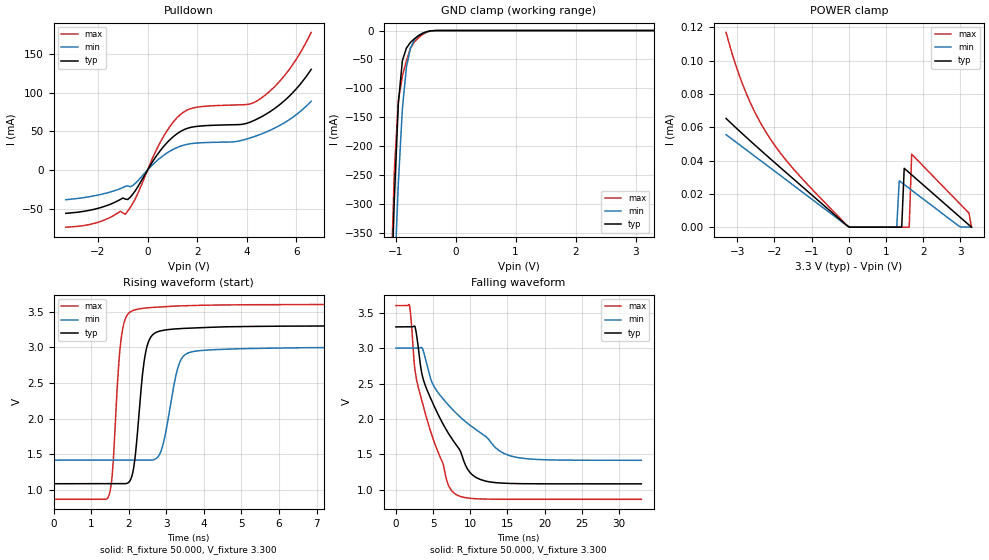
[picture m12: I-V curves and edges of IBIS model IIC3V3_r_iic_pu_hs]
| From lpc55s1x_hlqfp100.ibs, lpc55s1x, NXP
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|   Model IIC3V3_r_iic_pu_hs
[Model] IIC3V3_r_iic_pu_hs
Model_type I/O_open_drain
Polarity   Non-Inverting
Enable   Active-Low
Vinl =  0.990V
Vinh =  2.310V
Vmeas =  1.650V
Cref =  0.0F
Rref =  100.000
Vref =  3.3V
C_comp   2.434pF   2.433pF   2.440pF
C_comp_pulldown   1.615pF   1.554pF   1.667pF
C_comp_power_clamp   0.538pF   0.435pF   0.627pF
[Model Spec]
Vinh   2.310V   2.100V   2.520V
Vinl   0.990V   0.900V   1.080V
Vmeas   1.650V   1.500V   1.800V
Vref   3.3V   3.0V   3.6V
Cref   0.0F   0.0F   0.0F
Rref   100.000   100.000   100.000
[Temperature Range]   25.000   0.125k   -40.000
[Voltage Range]   3.300V   3.000V   3.600V
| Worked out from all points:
|   slope of the pulldown table from 0 to 0.495 V, typ, clamps not added: 20.4 ohm
|   GND clamp passes 1 mA (typ) near -0.43 V on its own axis
|   rising waveform, R_fixture 50.000, V_fixture 3.300: 20-80 % time 242ps typ, 336ps min, 194ps max; typ from 1.08 V to 3.3 V
|   falling waveform, R_fixture 50.000, V_fixture 3.300: 20-80 % time 5.56ns typ, 7.92ns min, 3.88ns max; typ from 3.3 V to 1.08 V
[Pulldown]
|Voltage   I(typ)   I(min)   I(max)
-3.3V     -56mA      -38.4mA    -73.87mA
-2.1V     -50.37mA   -33.07mA   -68.52mA
-1.1V     -38.15mA   -24.11mA   -53.37mA
-900mV    -37.61mA   -21.16mA   -57.18mA
-500mV    -26.92mA   -17.4mA    -37.43mA
500mV     24.51mA    15.34mA    35.14mA
1.2V      47.07mA    29.16mA    67.89mA
1.9V      55.94mA    34.55mA    80.54mA
3.8V      58.93mA    38.31mA    84.23mA
4.5V      67.15mA    45.39mA    91.04mA
5.6V      91.85mA    62.59mA    125mA
6.6V      130mA      88.72mA    177.8mA
[GND_clamp]
|Voltage   I(typ)   I(min)   I(max)
-3.3V     -10.05A    -9.18A     -11.33A
-1.089V   -516.5mA   -633.7mA   -475mA
-1.022V   -291.9mA   -436.3mA   -243.2mA
-955mV    -126mA     -264mA     -120.7mA
-888mV    -52.17mA   -135.6mA   -79.12mA
-821mV    -30.44mA   -63.69mA   -52.12mA
-754mV    -20.67mA   -30.69mA   -31.05mA
-687mV    -14.19mA   -15.97mA   -19.65mA
-553mV    -5.021mA   -4.512mA   -7.044mA
-419mV    -659.6uA   -714.3uA   -896.4uA
-285mV    -20.38uA   -37.42uA   -22.84uA
3.3V      0A         0A         0A
[POWER_clamp]
|Voltage   I(typ)   I(min)   I(max)
-3.3V     65.36uA    55.62uA    117.1uA
-2.797V   54.84uA    47.15uA    82.63uA
-2.194V   42.78uA    37.02uA    55.95uA
-50mV     976.9nA    858.9nA    1.15uA
1.29V     0A         0A         0A
1.357V    0A         27.85uA    0A
1.424V    0A         26.71uA    0A
1.491V    35.37uA    25.58uA    0A
1.625V    32.75uA    23.31uA    0A
1.692V    31.44uA    22.17uA    43.84uA
3.233V    1.309uA    0A         8.433uA
3.3V      0A         0A         0A
[Ramp]
| variable   typ   min   max
dV/dt_r   1.329/0.241n   0.951/0.336n   1.640/0.194n
dV/dt_f   1.329/5.558n   0.950/7.919n   1.640/3.880n
R_load = 50.000
[Rising Waveform]
R_fixture= 50.000
V_fixture= 3.300
V_fixture_min= 3.000
V_fixture_max= 3.600
|time   V(typ)   V(min)   V(max)
0s        1.085V     1.415V     866.6mV
1.467ns   1.085V     1.415V     908.4mV
1.83ns    1.084V     1.415V     3.23V
2.113ns   1.251V     1.415V     3.515V
2.317ns   2.334V     1.415V     3.542V
2.624ns   3.167V     1.417V     3.558V
2.908ns   3.237V     1.623V     3.567V
3.363ns   3.262V     2.794V     3.58V
3.91ns    3.275V     2.953V     3.589V
33ns      3.3V       3V         3.6V
[Falling Waveform]
R_fixture= 50.000
V_fixture= 3.300
V_fixture_min= 3.000
V_fixture_max= 3.600
|time   V(typ)   V(min)   V(max)
0s        3.3V       3V         3.6V
1.819ns   3.3V       3V         3.607V
2.49ns    3.313V     3V         2.757V
2.92ns    3.08V      3V         2.485V
3.941ns   2.476V     2.861V     2.08V
5.062ns   2.2V       2.471V     1.7V
7.82ns    1.677V     2.112V     954.1mV
12.21ns   1.12V      1.742V     869.5mV
16.65ns   1.088V     1.452V     866.9mV
33ns      1.085V     1.417V     866.6mV
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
